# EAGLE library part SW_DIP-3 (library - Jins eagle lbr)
DIP SWITCH
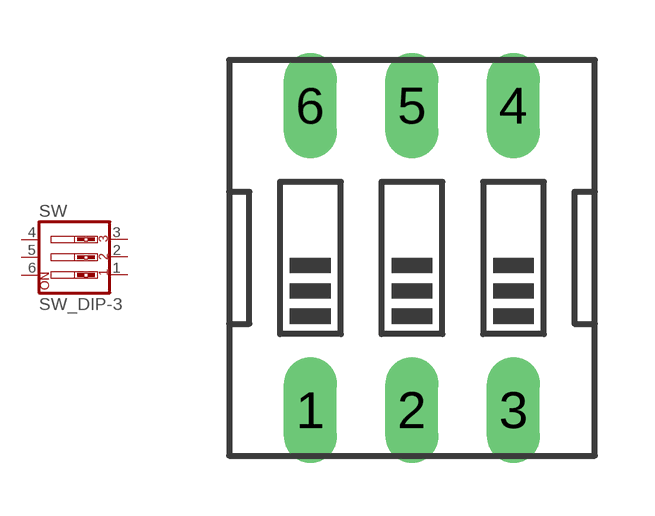
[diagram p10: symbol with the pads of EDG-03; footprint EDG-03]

Designator prefix SW

## SW_DIP-3  [EDG-03]
1  1  pas
2  2  pas
3  3  pas
4  4  pas
5  5  pas
6  6  pas

## Footprint EDG-03 (pad centres in mm)
DIP SWITCH
drill 0.813 long: 1 -2.54,-3.81; 2 0,-3.81; 3 2.54,-3.81; 4 2.54,3.81; 5 0,3.81; 6 -2.54,3.81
